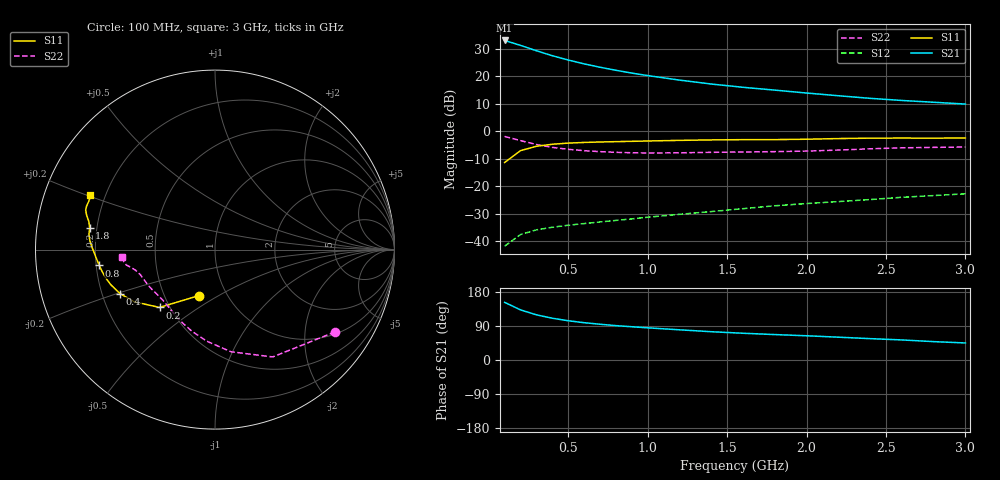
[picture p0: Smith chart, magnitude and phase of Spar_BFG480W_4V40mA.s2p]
! Filename: 440BFG480.001
! Title: BFG480W
! Bias: Vce=4V; Ic=40mA
! Company: NXP Semiconductors NL
! User: Quality&Reliability T&D
! Measure time: 10 Nov 1999 / 12:02:47
#  MHz  S  MA  R 50
! Freq  S11  S21  S12  S22  :
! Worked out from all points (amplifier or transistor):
!   20 points, 100 MHz to 3 GHz, reference 50 ohm
!   highest |S21| = 33.0 dB at 100 MHz (marker M1)
!   |S21| within 3 dB of that: start of sweep to 262.4 MHz
!   unconditionally stable (mu >= 1): 1.046 GHz to end of sweep
!   at 400 MHz: K = 0.59, MSG = 31.2 dB, |S12| = -34.8 dB
!   at 1.2 GHz: K = 1.04, MAG = 23.2 dB, |S12| = -30.2 dB
!   at 3 GHz: K = 1.07, MAG = 14.8 dB, |S12| = -22.7 dB
!   S11 on the Smith chart (normalised r, x): 100 MHz: 0.74, -0.41; 200 MHz: 0.44, -0.35; 400 MHz: 0.27, -0.20; 800 MHz: 0.21, -0.07; 1.8 GHz: 0.17, +0.08; 3 GHz: 0.14, +0.21
100  0.2722 -109.5  44.9 152.2  0.008201 64.6  0.8105 -34.5
200  0.4464 -133.8  36.58 132.3  0.01333 55.1  0.6791 -61.7
300  0.5358 -147.1  29.21 119.2  0.01622 50.7  0.5765 -81.0
400  0.5833 -155.2  23.72 110.2  0.0181 49.4  0.512 -95.2
500  0.6118 -161.2  19.81 103.6  0.01966 49.9  0.472 -106.0
600  0.6293 -165.6  16.87 98.5  0.02112 51.1  0.4459 -114.2
700  0.6411 -169.1  14.65 94.3  0.02258 53.1  0.4284 -120.8
800  0.6506 -172.2  12.89 90.8  0.02409 55.1  0.4163 -126.3
900  0.6594 -174.8  11.47 87.7  0.02567 57.5  0.4087 -131.1
1000  0.6686 -177.3  10.33 84.9  0.02753 59.2  0.4053 -135.4
1200  0.6863 178.7  8.55 79.7  0.03106 62.4  0.4078 -142.7
1400  0.6998 175.8  7.255 74.7  0.03487 64.9  0.4161 -148.1
1600  0.707 173.0  6.325 70.6  0.0394 67.2  0.4222 -152.2
1800  0.7089 170.1  5.623 67.1  0.04445 69.0  0.4285 -156.4
2000  0.7197 167.5  4.977 63.9  0.04874 70.7  0.4381 -161.2
2200  0.74 165.1  4.444 60.2  0.05296 71.4  0.4573 -165.5
2400  0.7532 163.1  3.986 56.4  0.05763 71.6  0.4822 -168.4
2600  0.7554 161.3  3.644 53.0  0.06344 71.6  0.5022 -170.2
2800  0.7531 159.0  3.381 48.5  0.06813 70.7  0.5121 -172.3
3000  0.7584 156.2  3.139 45.0  0.07333 70.4  0.5199 -175.4
